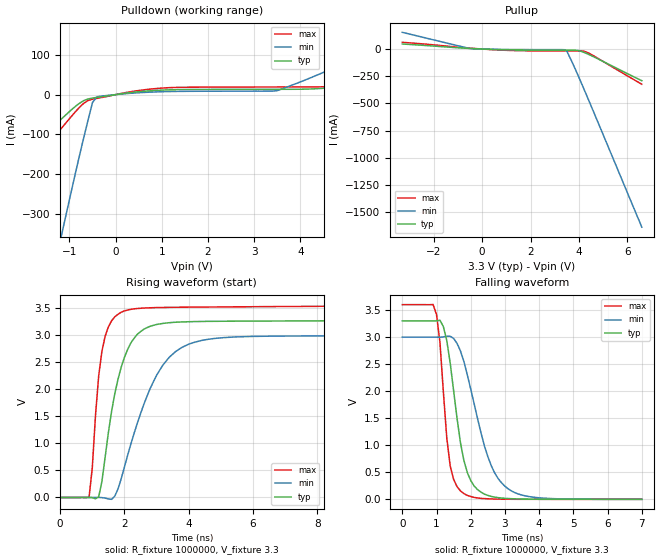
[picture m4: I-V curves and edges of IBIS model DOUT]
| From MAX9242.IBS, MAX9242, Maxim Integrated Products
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|   Model DOUT
[Model]   DOUT
Model_type   Output
|Signal   RxOUT[0:20]
|   typ   min   max
C_comp   2.9pF   2.7pF   3.2pF
[Temperature Range]   25.00   85.00   -40
[Voltage Range]   3.30V   3.00V   3.60V
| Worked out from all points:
|   slope of the pulldown table from 0 to 0.495 V, typ, clamps not added: 69 ohm
|   slope of the pullup table from 0 to 0.495 V, typ, clamps not added: 119 ohm
|   falling waveform, R_fixture 1000000, V_fixture 3.3: 20-80 % time 455ps typ, 756ps min, 278ps max; typ from 3.3 V to 0 V
|   rising waveform, R_fixture 1000000, V_fixture 3.3: 20-80 % time 644ps typ, 1.12ns min, 337ps max; typ from 0 V to 3.29 V
[Pulldown]
|Volts   I(typ)   I(min)   I(max)
-3.3V     -298.8mA   -1.486A    -365.9mA
-3.1V     -277.2mA   -1.379A    -340.7mA
-1.2V     -64.23mA   -368.3mA   -88.37mA
-1.1V     -53.21mA   -315.9mA   -74.39mA
-800mV    -23.22mA   -162mA     -34.15mA
-600mV    -11.01mA   -65.76mA   -14.9mA
-500mV    -8.581mA   -19.61mA   -11.51mA
-400mV    -6.871mA   -5.258mA   -9.344mA
1V        11.32mA    7.284mA    16.37mA
3.5V      13.37mA    10.07mA    19.16mA
4.8V      18.73mA    70.85mA    22.28mA
6.6V      45.6mA     167mA      56.9mA
[Pullup]
|Volts   I(typ)   I(min)   I(max)
-3.3V     46.2mA     153.5mA    61.51mA
-500mV    5.174mA    4.736mA    8.165mA
1.2V      -7.789mA   -4.67mA    -13.41mA
3.4V      -10.41mA   -6.529mA   -18.04mA
3.5V      -10.46mA   -19.88mA   -18.12mA
4V        -15.12mA   -260.2mA   -18.45mA
4.3V      -39.38mA   -415.7mA   -26.56mA
6.6V      -291.4mA   -1.638A    -323.8mA
[Ramp]
|Variable   typ   min   max
dV/dt_r  1.89/0.62n  1.79/1.12n  2.16/0.34n
dV/dt_f  1.97/0.44n  1.77/0.74n  2.07/0.26n
R_load=1000000
[Falling Waveform]
R_fixture = 1000000 |output open
C_fixture = 0.0
V_fixture = 3.3
V_fixture_min = 3.0
V_fixture_max = 3.6
|Time   V(typ)   V(min)   V(max)
0s        3.3V       2.999V     3.6V
1ns       3.301V     2.999V     3.417V
1.1ns     3.312V     2.998V     2.904V
1.2ns     3.195V     3.003V     1.988V
1.4ns     2.519V     3.016V     617.5mV
1.7ns     1.047V     2.743V     156.3mV
2.1ns     246.6mV    1.766V     34.55mV
2.5ns     72.63mV    790.3mV    9.796mV
3ns       18.59mV    241.8mV    2.458mV
7ns       14.34uV    139.2uV    12.21uV
[Rising Waveform]
R_fixture = 1000000 | output open
C_fixture = 0.0
V_fixture = 3.3
V_fixture_min = 3.0
V_fixture_max = 3.6
|Time   V(typ)   V(min)   V(max)
0s        0V         0V         0V
900ps     634.4uV    -119.9uV   5.618mV
1ns       -4.415mV   183.8uV    546.6mV
1.2ns     11.5mV     439.9uV    2.252V
1.3ns     298.5mV    -2.818mV   2.705V
1.7ns     1.919V     23.83mV    3.343V
2ns       2.594V     561.9mV    3.453V
3ns       3.202V     2.26V      3.515V
4.4ns     3.258V     2.906V     3.525V
20ns      3.287V     2.994V     3.572V
